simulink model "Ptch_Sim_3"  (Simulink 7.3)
settings: Solver=ode45  StartTime=0.0  StopTime=250  RelTol=1e-3
InitFcn:
  | init
StopFcn:
  | Pl
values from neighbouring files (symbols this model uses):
  Aac = [    [actuator.m]
  Aes = [    [estimator.m]
  Bac = [    [actuator.m]
  Bes = [    [estimator.m]
  Cac = [    [actuator.m]
  Ces = [    [estimator.m]
  d2r = pi/180    (= 0.0174532925199)    [init.m]    (also in run.m; LQR_Des.m)
  Dac = [    [actuator.m]
  Des = [    [estimator.m]
  r2d = 1/d2r    (= 57.2957795131)    [init.m]    (also in Pl.m; run.m; LQR_Des.m)
undefined symbols (not defined in the file or in its folder): Apc, Avf, Bpc, Bvf, Cpc, Cvf, Dpc, Dvf

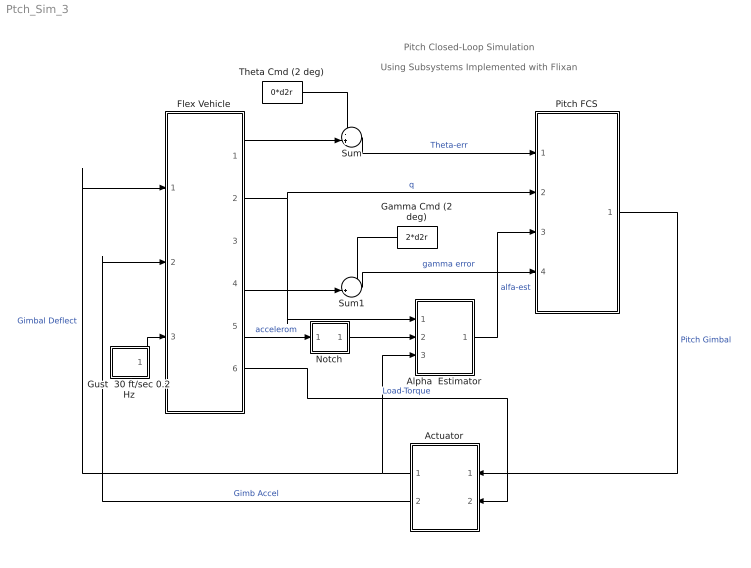
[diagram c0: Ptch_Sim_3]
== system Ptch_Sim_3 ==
  note: Pitch Closed-Loop Simulation
  note: Using Subsystems Implemented with Flixan
  Actuator : Subsystem
  Alpha  Estimator : Subsystem
  Flex Vehicle : Subsystem
  Gamma Cmd (2 deg) : Constant  Value=2*d2r  OutDataType=sfix(16)  OutScaling=2^0
  Gust  30 ft/sec 0.2 Hz : Subsystem
  Notch : Subsystem
  Pitch FCS : Subsystem
  Sum : Sum  Inputs=-+|  OutDataType=sfix(16)  OutScaling=2^0
  Sum1 : Sum  Inputs=-+|  OutDataType=sfix(16)  OutScaling=2^0
  Theta Cmd (2 deg) : Constant  Value=0*d2r  OutDataType=sfix(16)  OutScaling=2^0
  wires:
  Flex Vehicle/2(q-flex) -> Alpha  Estimator/1(q-flx), Pitch FCS/2(q)  "q"
  Flex Vehicle/1(theta) -> Sum/2
  Sum/1 -> Pitch FCS/1(Theta)  "Theta-err"
  Flex Vehicle/4(gama) -> Sum1/2
  Sum1/1 -> Pitch FCS/4(gamma)  "gamma error"
  Alpha  Estimator/1(alphat) -> Pitch FCS/3(alpha)  "alfa-est"
  Flex Vehicle/5(Zdd-flex) -> Notch/1(In)  "accelerom"
  Gust  30 ft/sec 0.2 Hz/1(Vgust) -> Flex Vehicle/3(Gust)
  Gamma Cmd (2 deg)/1 -> Sum1/1
  Theta Cmd (2 deg)/1 -> Sum/1
  Notch/1(Ou) -> Alpha  Estimator/2(Zdd)
  Pitch FCS/1(delta) -> Actuator/1(Dyc)  "Pitch Gimbal"
  Actuator/1(Dy) -> Flex Vehicle/1(Dy), Alpha  Estimator/3(delta)  "Gimbal Deflect"
  Actuator/2(Dy_dd) -> Flex Vehicle/2(Dy_dd)  "Gimb Accel"
  Flex Vehicle/6(TLy) -> Actuator/2(TLy)  "Load-Torque"

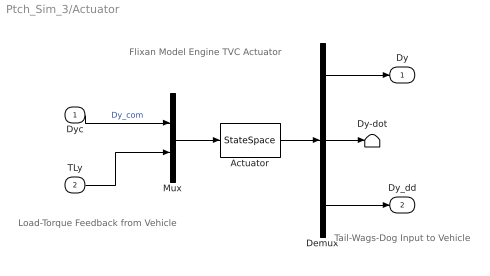
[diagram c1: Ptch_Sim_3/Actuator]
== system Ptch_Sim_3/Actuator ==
  note: Flixan Model Engine TVC Actuator
  note: Load-Torque Feedback from Vehicle
  note: Tail-Wags-Dog Input to Vehicle
  Dyc : Inport  OutDataType=sfix(16)  OutScaling=2^0
  TLy : Inport  Port=2  OutDataType=sfix(16)  OutScaling=2^0
  Actuator : StateSpace  A=Aac  B=Bac  C=Cac  D=Dac
  Demux : Demux  Outputs=3
  Dy-dot : Terminator
  Mux : Mux  Inputs=2
  Dy : Outport  OutDataType=sfix(16)  OutScaling=2^0
  Dy_dd : Outport  Port=2  OutDataType=sfix(16)  OutScaling=2^0
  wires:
  TLy/1 -> Mux/2
  Demux/3 -> Dy_dd/1
  Demux/1 -> Dy/1
  Dyc/1 -> Mux/1  "Dy_com"
  Demux/2 -> Dy-dot/1
  Actuator/1 -> Demux/1
  Mux/1 -> Actuator/1

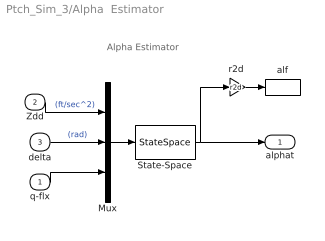
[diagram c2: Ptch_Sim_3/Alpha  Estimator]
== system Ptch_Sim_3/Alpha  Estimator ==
  note: Alpha Estimator
  q-flx : Inport  OutDataType=sfix(16)  OutScaling=2^0
  Zdd : Inport  Port=2  OutDataType=sfix(16)  OutScaling=2^0
  delta : Inport  Port=3  OutDataType=sfix(16)  OutScaling=2^0
  Mux : Mux  Inputs=3
  State-Space : StateSpace  A=Aes  B=Bes  C=Ces  D=Des
  alf : ToWorkspace  VariableName=alphat  SampleTime=-1  SaveFormat=Array
  "r2d " : Gain  Gain=r2d  ParameterDataType=sfix(16)  ParameterScaling=2^0  OutDataType=sfix(16)  OutScaling=2^0
  alphat : Outport  OutDataType=sfix(16)  OutScaling=2^0
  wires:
  State-Space/1 -> alphat/1, "r2d "/1
  Mux/1 -> State-Space/1
  Zdd/1 -> Mux/1  "(ft/sec^2)"
  delta/1 -> Mux/2  "(rad)"
  q-flx/1 -> Mux/3
  "r2d "/1 -> alf/1

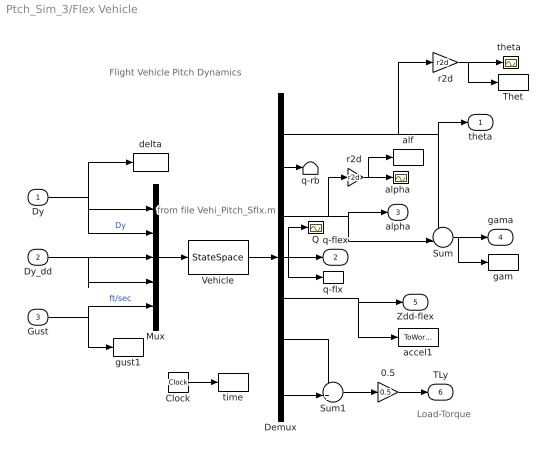
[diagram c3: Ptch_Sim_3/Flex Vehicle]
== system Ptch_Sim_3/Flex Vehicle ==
  note: Load-Torque
  note: from file Vehi_Pitch_Sflx.m
  note: Flight Vehicle Pitch Dynamics
  Dy : Inport  OutDataType=sfix(16)  OutScaling=2^0
  Dy_dd : Inport  Port=2  OutDataType=sfix(16)  OutScaling=2^0
  Gust : Inport  Port=3  OutDataType=sfix(16)  OutScaling=2^0
  0.5 : Gain  Gain=0.5  ParameterDataType=sfix(16)  ParameterScaling=2^0  OutDataType=sfix(16)  OutScaling=2^0
  Clock : Clock
  Demux : Demux  Outputs=7
  Mux : Mux  Inputs=5
  Q : Scope
  Sum : Sum  Inputs=+-|  OutDataType=sfix(16)  OutScaling=2^0
  Sum1 : Sum  Inputs=++|  OutDataType=sfix(16)  OutScaling=2^0
  Thet : ToWorkspace  VariableName=theta  SampleTime=-1  SaveFormat=Array
  Vehicle : StateSpace  A=Avf  B=Bvf  C=Cvf  D=Dvf
  accel1 : ToWorkspace  VariableName=accel  SampleTime=-1  SaveFormat=Array
  alf : ToWorkspace  VariableName=alpha  SampleTime=-1  SaveFormat=Array
  "alpha  " : Scope
  delta : ToWorkspace  VariableName=delta  SampleTime=-1  SaveFormat=Array
  gam : ToWorkspace  VariableName=gama  SampleTime=-1  SaveFormat=Array
  gust1 : ToWorkspace  VariableName=Gust  SampleTime=-1  SaveFormat=Array
  q-flx : ToWorkspace  VariableName=q  SampleTime=-1  SaveFormat=Array
  q-rb : Terminator
  r2d : Gain  Gain=r2d  ParameterDataType=sfix(16)  ParameterScaling=2^0  OutDataType=sfix(16)  OutScaling=2^0
  "r2d " : Gain  Gain=r2d  ParameterDataType=sfix(16)  ParameterScaling=2^0  OutDataType=sfix(16)  OutScaling=2^0
  "theta " : Scope
  time : ToWorkspace  VariableName=time  SampleTime=-1  SaveFormat=Array
  theta : Outport  OutDataType=sfix(16)  OutScaling=2^0
  q-flex : Outport  Port=2  OutDataType=sfix(16)  OutScaling=2^0
  alpha : Outport  Port=3  OutDataType=sfix(16)  OutScaling=2^0
  gama : Outport  Port=4  OutDataType=sfix(16)  OutScaling=2^0
  Zdd-flex : Outport  Port=5  OutDataType=sfix(16)  OutScaling=2^0
  TLy : Outport  Port=6  OutDataType=sfix(16)  OutScaling=2^0
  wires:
  Sum1/1 -> 0.5/1
  0.5/1 -> TLy/1
  "r2d "/1 -> alf/1, "alpha  "/1
  r2d/1 -> Thet/1, "theta "/1
  Clock/1 -> time/1
  Demux/2 -> q-rb/1
  Demux/4 -> Q/1, q-flx/1, q-flex/1
  Sum/1 -> gam/1, gama/1
  Demux/6 -> Sum1/1
  Demux/7 -> Sum1/2
  Demux/5 -> accel1/1, Zdd-flex/1
  Demux/3 -> "r2d "/1, alpha/1, Sum/2
  Demux/1 -> r2d/1, Sum/1, theta/1
  Dy_dd/1 -> Mux/4, Mux/3
  Gust/1 -> gust1/1, Mux/5  "ft/sec"
  Dy/1 -> delta/1, Mux/2, Mux/1  "Dy"
  Vehicle/1 -> Demux/1
  Mux/1 -> Vehicle/1

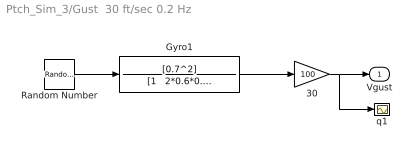
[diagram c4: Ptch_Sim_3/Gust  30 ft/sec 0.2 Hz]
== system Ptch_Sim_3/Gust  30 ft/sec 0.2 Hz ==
  30 : Gain  Gain=100  ParameterDataType=sfix(16)  ParameterScaling=2^0  OutDataType=sfix(16)  OutScaling=2^0
  Gyro1 : TransferFcn  Numerator=[0.7^2]  Denominator="[1   2*0.6*0.7   0.7^2]"
  Random Number : RandomNumber  Seed=-2  SampleTime=0
  q1 : Scope
  Vgust : Outport  OutDataType=sfix(16)  OutScaling=2^0
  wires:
  30/1 -> q1/1, Vgust/1
  Gyro1/1 -> 30/1
  Random Number/1 -> Gyro1/1

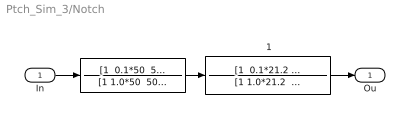
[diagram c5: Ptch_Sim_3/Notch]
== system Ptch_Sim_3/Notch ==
  In : Inport
  " " : TransferFcn  Numerator="[1  0.1*50  50^2]"  Denominator="[1 1.0*50  50^2]"
  " 1" : TransferFcn  Numerator="[1  0.1*21.2  21.2^2]"  Denominator="[1 1.0*21.2  21.2^2]"
  Ou : Outport
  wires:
  " "/1 -> " 1"/1
  In/1 -> " "/1
  " 1"/1 -> Ou/1

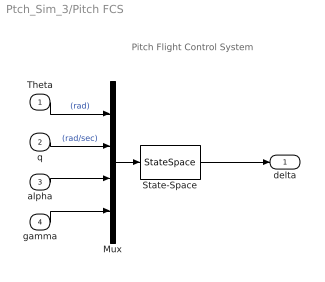
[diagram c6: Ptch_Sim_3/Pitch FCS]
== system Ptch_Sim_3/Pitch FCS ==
  note: Pitch Flight Control System
  Theta : Inport  OutDataType=sfix(16)  OutScaling=2^0
  q : Inport  Port=2  OutDataType=sfix(16)  OutScaling=2^0
  alpha : Inport  Port=3  OutDataType=sfix(16)  OutScaling=2^0
  gamma : Inport  Port=4  OutDataType=sfix(16)  OutScaling=2^0
  Mux : Mux
  State-Space : StateSpace  A=Apc  B=Bpc  C=Cpc  D=Dpc
  delta : Outport  OutDataType=sfix(16)  OutScaling=2^0
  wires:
  State-Space/1 -> delta/1
  Mux/1 -> State-Space/1
  Theta/1 -> Mux/1  "(rad)"
  q/1 -> Mux/2  "(rad/sec)"
  alpha/1 -> Mux/3
  gamma/1 -> Mux/4
